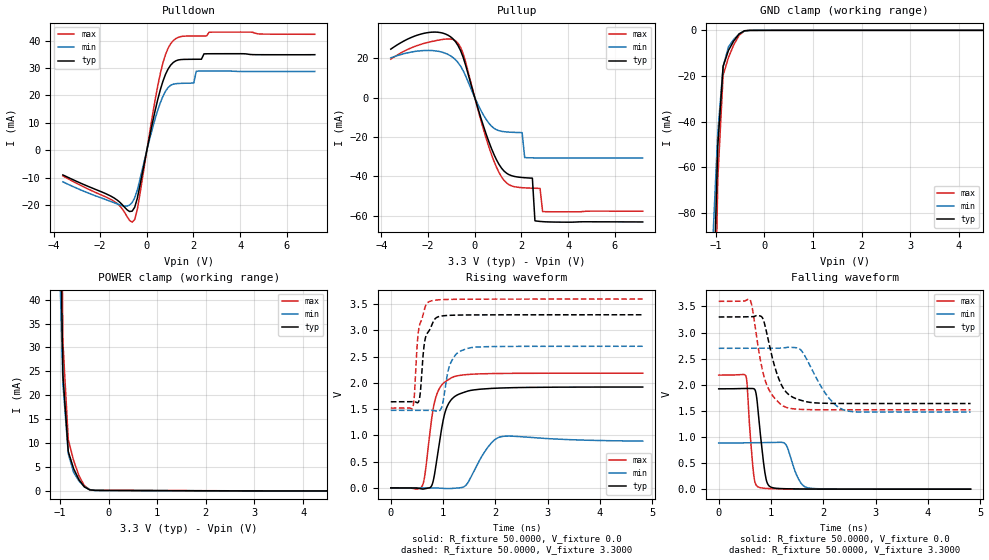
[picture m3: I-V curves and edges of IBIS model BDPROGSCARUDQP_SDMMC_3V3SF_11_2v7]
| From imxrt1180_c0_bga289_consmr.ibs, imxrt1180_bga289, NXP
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[Model]  BDPROGSCARUDQP_SDMMC_3V3SF_11_2v7
|   Model BDPROGSCARUDQP_SDMMC_3V3SF_11_2v7
| This model was characterised for following simulation conditions:
| External (pad) voltage:
|   - Typ: 3.3V,   - Min: 2.7V,   - Max: 3.6V
| Library cells for typ/min/max conditions are connected as defined below:
|  IO - External Pad
|  A - Core Input
|  EN - Output Buffer Enable
|  ASRCN3V3[0] - REFH3V3
|  ASRCN3V3[1] - REFH3V3 REFH3V3 gnde
|  ASRCN3V3[2] - gnde REFH3V3 gnde
|  ASRCN3V3[3] - gnde REFH3V3 gnde
|  ASRCP3V3[0] - vdde3v3 REFL3V3 REFL3V3
|  ASRCP3V3[1] - vdde3v3 REFL3V3 vdde3v3
|  ASRCP3V3[2] - REFL3V3 REFL3V3 vdde3v3
|  ASRCP3V3[3] - REFL3V3 REFL3V3 vdde3v3
|  IOGC - NC
|  PDRV - vdd
|  PSW - vdd
|  REFH3V3 - REFH3V3
|  REFL3V3 - REFL3V3
|  ZI - NC
|  gnd - gnd
|  gnde - gnde
|  vdd - vdd
|  vdde3v3 - vdde3v3
| All other pins connected to ground
Model_type I/O
Polarity   Non-Inverting
Enable   Active-Low
Vinl =   0.6750V
Vinh =   2.2500V
Vmeas =  1.6500V
Cref =   30.0000pF
Rref =   1.0000M
Vref =   3.3000V
C_comp   2.1236pF   2.1010pF   2.1446pF
|C_comp_pullup   0.3619pF   0.3769pF   0.3519pF
|C_comp_pulldown   0.6265pF   0.6593pF   0.5997pF
[Model Spec]
| variable   typ   min   max
Vinh   2.0625V   1.6875V   2.2500V
Vinl   0.8250V   0.6750V   0.9000V
[Temperature Range]   25.0000   0.1050k   -20.0000
[Voltage Range]   3.3000V   2.7000V   3.6000V
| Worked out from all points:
|   slope of the pulldown table from 0 to 0.495 V, typ, clamps not added: 25.5 ohm
|   slope of the pullup table from 0 to 0.495 V, typ, clamps not added: 26.4 ohm
|   GND clamp passes 1 mA (typ) near -0.48 V on its own axis
|   POWER clamp passes 1 mA (typ) near -0.51 V on its own axis
|   rising waveform, R_fixture 50.0000, V_fixture 0.0: 20-80 % time 215ps typ, 293ps min, 191ps max; typ from 0 V to 1.92 V
|   rising waveform, R_fixture 50.0000, V_fixture 3.3000: 20-80 % time 135ps typ, 171ps min, 120ps max; typ from 1.64 V to 3.3 V
|   falling waveform, R_fixture 50.0000, V_fixture 0.0: 20-80 % time 124ps typ, 192ps min, 93.1ps max; typ from 1.92 V to 0 V
|   falling waveform, R_fixture 50.0000, V_fixture 3.3000: 20-80 % time 290ps typ, 427ps min, 260ps max; typ from 3.3 V to 1.64 V
[Pulldown]
|Voltage   I(typ)   I(min)   I(max)
-3.6V     -8.96mA    -11.48mA   -9.321mA
-1.4V     -17.38mA   -19.1mA    -18.58mA
-630mV    -22.15mA   -19.01mA   -26.18mA
-410mV    -17.5mA    -14.49mA   -21.62mA
250mV     10.41mA    8.306mA    13.2mA
580mV     22.14mA    17.4mA     28.06mA
800mV     27.69mA    21.55mA    34.89mA
1.13V     32mA       24.11mA    39.96mA
2.01V     33.18mA    24.51mA    41.67mA
2.12V     33.19mA    28.85mA    41.67mA
2.45V     35.15mA    28.88mA    41.69mA
7.2V      34.85mA    28.74mA    42.29mA
[Pullup]
|Voltage   I(typ)   I(min)   I(max)
-3.6V     24.55mA    20.12mA    19.48mA
-1.93V    33.06mA    23.88mA    28.19mA
-830mV    28.38mA    19.21mA    28.82mA
-500mV    20.5mA     13.69mA    22.35mA
1.04V     -33.9mA    -16.82mA   -38mA
2.03V     -40.55mA   -17.78mA   -45.71mA
2.14V     -40.66mA   -30.44mA   -45.79mA
2.47V     -40.88mA   -30.58mA   -45.96mA
2.58V     -62.51mA   -30.6mA    -46mA
2.8V      -62.83mA   -30.63mA   -46.07mA
2.91V     -62.93mA   -30.64mA   -57.84mA
7.2V      -63.09mA   -30.66mA   -57.63mA
[GND_clamp]
|Voltage   I(typ)   I(min)   I(max)
-3.6V     -5.131A    -2.966A    -8.406A
-1.07V    -134.2mA   -96.06mA   -200.7mA
-960mV    -50.84mA   -45.02mA   -65.28mA
-850mV    -15.74mA   -15.88mA   -19.63mA
-740mV    -8.808mA   -7.25mA    -11.89mA
-630mV    -4.596mA   -3.893mA   -6.316mA
-520mV    -1.551mA   -1.564mA   -2.126mA
-410mV    -182.3uA   -311.4uA   -219.4uA
-190mV    -16.94uA   -12.12uA   -23.77uA
7.2V      0A         0A         0A
[POWER_clamp]
|Voltage   I(typ)   I(min)   I(max)
-3.6V     5.01A      2.849A     8.324A
-1.05V    90.64mA    63.65mA    144.9mA
-940mV    24.29mA    22.45mA    31.15mA
-830mV    8.246mA    7.775mA    10.76mA
-720mV    4.663mA    3.883mA    6.37mA
-610mV    2.344mA    2.086mA    3.186mA
-500mV    850.8uA    898.3uA    1.111mA
-390mV    222uA      282.9uA    270.2uA
-170mV    103uA      69.45uA    142.4uA
7.2V      0A         0A         0A
[Ramp]
| variable   typ   min   max
dV/dt_r  1.1530/0.2150n   0.5348/0.2933n   1.3109/0.1906n
dV/dt_f  0.9946/0.2895n   0.7323/0.4268n   1.2465/0.2597n
R_load = 50.0000
[Rising Waveform]
R_fixture= 50.0000
V_fixture= 0.0
V_fixture_min= 0.0
V_fixture_max= 0.0
|time   V(typ)   V(min)   V(max)
0s        169.4uV    118.1uV    212.9uV
598.6ps   -21.02mV   164.9uV    32.03mV
654.5ps   -15.23mV   173.9uV    262.2mV
775.8ps   30.64mV    39.56uV    1.27V
867.8ps   453.8mV    -1.438mV   1.747V
1.018ns   1.363V     -10.42mV   2.005V
1.173ns   1.698V     -8.769mV   2.105V
1.434ns   1.833V     47.37mV    2.158V
2.107ns   1.903V     975mV      2.181V
4.82ns    1.922V     891.4mV    2.185V
[Rising Waveform]
R_fixture= 50.0000
V_fixture= 3.3000
V_fixture_min= 2.7000
V_fixture_max= 3.6000
|time   V(typ)   V(min)   V(max)
0s        1.641V     1.478V     1.52V
417.9ps   1.643V     1.478V     1.526V
449.7ps   1.643V     1.478V     1.744V
533.6ps   1.647V     1.478V     3.019V
640.1ps   2.737V     1.478V     3.392V
734.8ps   2.997V     1.479V     3.549V
956.5ps   3.272V     1.498V     3.586V
1.137ns   3.289V     2.364V     3.592V
1.457ns   3.295V     2.654V     3.595V
4.82ns    3.298V     2.699V     3.598V
[Falling Waveform]
R_fixture= 50.0000
V_fixture= 0.0
V_fixture_min= 0.0
V_fixture_max= 0.0
|time   V(typ)   V(min)   V(max)
0s        1.922V     884.6mV    2.185V
520.5ps   1.929V     888.2mV    2.166V
663.4ps   1.926V     890mV      328.4mV
758.9ps   1.444V     890.4mV    40.32mV
891ps     273.5mV    892.7mV    15.47mV
1.01ns    34.43mV    895.5mV    9.226mV
1.28ns    8.106mV    860.8mV    3.791mV
1.51ns    4.299mV    227.1mV    1.959mV
1.694ns   2.706mV    28.45mV    1.203mV
4.82ns    169.5uV    153.6uV    212.8uV
[Falling Waveform]
R_fixture= 50.0000
V_fixture= 3.3000
V_fixture_min= 2.7000
V_fixture_max= 3.6000
|time   V(typ)   V(min)   V(max)
0s        3.298V     2.699V     3.598V
599.7ps   3.301V     2.699V     3.626V
809.3ps   3.312V     2.699V     2.412V
889.7ps   3.118V     2.7V       2.081V
1.088ns   2.293V     2.7V       1.724V
1.258ns   1.9V       2.709V     1.58V
1.576ns   1.701V     2.661V     1.527V
2.044ns   1.645V     1.832V     1.521V
2.397ns   1.641V     1.517V     1.52V
4.82ns    1.641V     1.478V     1.52V
